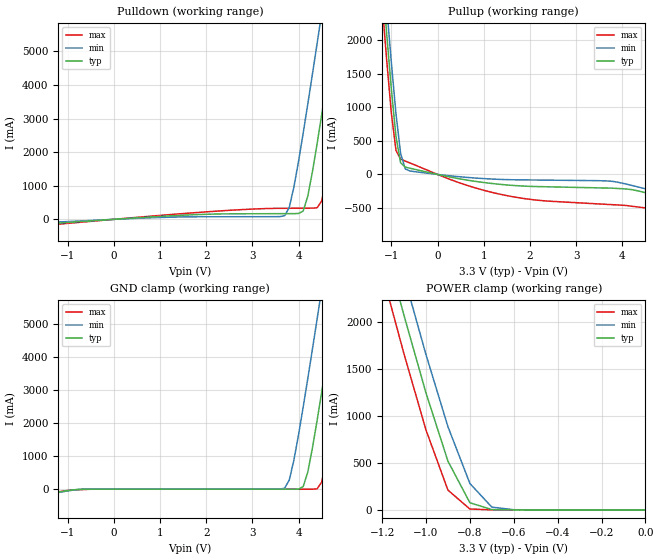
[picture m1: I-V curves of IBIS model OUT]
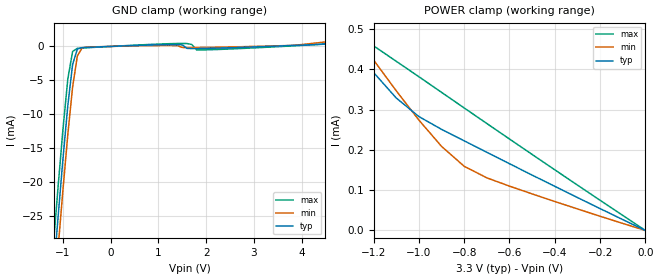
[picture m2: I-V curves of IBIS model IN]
|   TEXAS INSTRUMENTS INCORPORATED
|   Standard Linear and Logic
|   IBIS Model of SN74ALVCH16334
|   16-BIT Universal Bus Driver with 3-state outputs
|   48-pin DGG, DGV, or DL Package
[IBIS Ver]   2.1
[Comment char]  |_char
[File Name]   alvch16334.ibs
[File Rev]   2.0
[Date]   8/1/97
[Source]   File originated at Texas Instruments, Inc.
[Notes]   The following is an IBIS list for the ALVCH16334.
|   - This file may be incomplete or may not be fully compliant
|   with the IBIS specification. It will be replaced with a
|   version that is IBIS Revision 3.2 compliant and is complete
|   and accurate.  Please email all questions and comments to
|   sllibis@ti.com.
|   - All test data contained in this file are derived from
|   hspice(tm) simulations.
|   - File created by Ramzi Ammar, SLL Applications
[Disclaimer]
* Property of Texas Instruments Incorporated.  Unauthorized *
* reproduction and/or distribution is strictly prohibited. *
* This product is protected under copyright law. *
* Created 1997, (C) Copyright 1997, Texas Instruments Inc., *
* All Rights Reserved *
* UNLESS THERE IS A SIGNED, WRITTEN AGREEMENT TO THE *
* CONTRARY, TEXAS INSTRUMENTS ("TI") IS PROVIDING THE IBIS *
* MODELS "AS IS" AND WITHOUT ANY WARRANTY, EXPRESSED OR *
* IMPLIED.  TI assumes no liability for: *
* 1) the accuracy of the IBIS models provided to your *
* company; *
* 2) the proper functioning of these IBIS models in your *
* design or for any resulting applications; or *
* 3) infringement of patents, copyrights or intellectual *
* property rights resulting from your use of these *
* IBIS models. *
* TI provides IBIS Models as a service to our customers. *
* You and your company shall not distribute, sell or give *
* these models to anyone else without prior written *
* permission from TI. *
* TI reserves the right to make changes to our products or *
* to discontinue any semiconductor product or service *
* without notice, and advises our customers to obtain the *
* latest version of relevant information to verify, before *
* placing orders, that the information being relied on is *
* current. *
* Please be aware that your receipt and use of the IBIS *
* information provided shall serve as acceptance of these *
* terms and conditions.  If you do not accept these terms, *
* you should return or destroy the IBIS models and any *
* other accompanying information immediately. *
[Component]   ALVCH16334_DGG
[Manufacturer]  Texas Instruments, Inc.
[Package]
|   typ   min   max
R_pkg   0.056   0.039   0.068
L_pkg   3.39nH   3.078nH   3.995nH
C_pkg   0.52pF   0.414pF   0.668pF
[Pin]   signal_name   model_name   R_pin   L_pin   C_pin
1   OE_BAR   NC   0.039   3.987nH   0.654pF
2   Y1   OUT   0.047   3.725nH   0.659pF
3   Y2   OUT   0.059   3.692nH   0.604pF
4   GND   GND   0.068   3.675nH   0.606pF
5   Y3   OUT   0.055   3.473nH   0.547pF
6   Y4   OUT   0.056   3.402nH   0.497pF
7   VCC   POWER   0.057   3.3nH   0.492pF
8   Y5   OUT   0.056   3.189nH   0.455pF
9   Y6   OUT   0.058   3.154nH   0.449pF
10   GND   GND   0.058   3.094nH   0.436pF
11   Y7   OUT   0.058   3.078nH   0.424pF
12   Y8   OUT   0.06   3.081nH   0.414pF
13   Y9   OUT   0.061   3.097nH   0.416pF
14   Y10   OUT   0.06   3.126nH   0.427pF
15   GND   GND   0.061   3.158nH   0.44pF
16   Y11   OUT   0.058   3.173nH   0.45pF
17   Y12   OUT   0.056   3.189nH   0.455pF
18   VCC   POWER   0.056   3.265nH   0.49pF
19   Y13   OUT   0.054   3.322nH   0.492pF
20   Y14   OUT   0.052   3.388nH   0.544pF
21   GND   GND   0.064   3.591nH   0.605pF
22   Y15   OUT   0.059   3.677nH   0.612pF
23   Y16   OUT   0.046   3.678nH   0.668pF
24   NC   NC   0.041   3.979nH   0.659pF
25   LE_BAR   NC   0.04   3.995nH   0.658pF
26   A16   IN   0.046   3.69nH   0.662pF
27   A15   IN   0.057   3.649nH   0.602pF
28   GND   GND   0.066   3.615nH   0.602pF
29   A14   IN   0.055   3.447nH   0.547pF
30   A13   IN   0.054   3.326nH   0.492pF
31   VCC   POWER   0.055   3.239nH   0.488pF
32   A12   IN   0.056   3.183nH   0.454pF
33   A11   IN   0.057   3.144nH   0.447pF
34   GND   GND   0.058   3.099nH   0.436pF
35   A10   IN   0.059   3.086nH   0.425pF
36   A9   IN   0.06   3.081nH   0.414pF
37   A8   IN   0.061   3.097nH   0.415pF
38   A7   IN   0.06   3.119nH   0.427pF
39   GND   GND   0.06   3.144nH   0.439pF
40   A6   IN   0.056   3.13nH   0.446pF
41   A5   IN   0.057   3.208nH   0.456pF
42   VCC   POWER   0.056   3.247nH   0.487pF
43   A4   IN   0.054   3.328nH   0.491pF
44   A3   IN   0.053   3.413nH   0.546pF
45   GND   GND   0.066   3.609nH   0.606pF
46   A2   IN   0.058   3.689nH   0.607pF
47   A1   IN   0.047   3.727nH   0.662pF
48   CLK   NC   0.04   3.978nH   0.655pF
[Component]   ALVCH16334_DGV
[Manufacturer]  Texas Instruments, Inc.
[Package]
|   typ   min   max
R_pkg   0.063   0.043   0.09
L_pkg   3.077nH   2.377nH   4.305nH
C_pkg   0.387pF   0.281pF   0.565pF
[Pin]   signal_name   model_name   R_pin   L_pin   C_pin
1   OE_BAR   NC   0.082   4.277nH   0.562pF
2   Y1   OUT   0.09   4.02nH   0.554pF
3   Y2   OUT   0.087   3.719nH   0.478pF
4   GND   GND   0.087   3.456nH   0.417pF
5   Y3   OUT   0.076   3.207nH   0.411pF
6   Y4   OUT   0.044   2.929nH   0.39pF
7   VCC   POWER   0.046   2.803nH   0.335pF
8   Y5   OUT   0.047   2.683nH   0.321pF
9   Y6   OUT   0.048   2.579nH   0.311pF
10   GND   GND   0.049   2.505nH   0.302pF
11   Y7   OUT   0.048   2.4nH   0.289pF
12   Y8   OUT   0.051   2.4nH   0.283pF
13   Y9   OUT   0.051   2.4nH   0.283pF
14   Y10   OUT   0.05   2.433nH   0.291pF
15   GND   GND   0.048   2.46nH   0.298pF
16   Y11   OUT   0.048   2.585nH   0.312pF
17   Y12   OUT   0.046   2.652nH   0.319pF
18   VCC   POWER   0.045   2.787nH   0.336pF
19   Y13   OUT   0.046   2.962nH   0.394pF
20   Y14   OUT   0.074   3.208nH   0.409pF
21   GND   GND   0.087   3.488nH   0.417pF
22   Y15   OUT   0.087   3.741nH   0.478pF
23   Y16   OUT   0.089   3.99nH   0.546pF
24   NC   NC   0.084   4.305nH   0.557pF
25   LE_BAR   NC   0.082   4.286nH   0.565pF
26   A16   IN   0.086   3.933nH   0.554pF
27   A15   IN   0.086   3.699nH   0.475pF
28   GND   GND   0.089   3.522nH   0.42pF
29   A14   IN   0.079   3.234nH   0.413pF
30   A13   IN   0.043   2.88nH   0.385pF
31   VCC   POWER   0.045   2.779nH   0.332pF
32   A12   IN   0.045   2.636nH   0.317pF
33   A11   IN   0.047   2.553nH   0.309pF
34   GND   GND   0.048   2.468nH   0.298pF
35   A10   IN   0.05   2.424nH   0.29pF
36   A9   IN   0.05   2.377nH   0.281pF
37   A8   IN   0.05   2.387nH   0.281pF
38   A7   IN   0.05   2.431nH   0.29pF
39   GND   GND   0.048   2.475nH   0.299pF
40   A6   IN   0.048   2.557nH   0.309pF
41   A5   IN   0.047   2.671nH   0.319pF
42   VCC   POWER   0.046   2.804nH   0.334pF
43   A4   IN   0.044   2.935nH   0.39pF
44   A3   IN   0.074   3.203nH   0.412pF
45   GND   GND   0.085   3.444nH   0.416pF
46   A2   IN   0.085   3.723nH   0.477pF
47   A1   IN   0.09   4.012nH   0.547pF
48   CLK   NC   0.083   4.288nH   0.558pF
[Component]   ALVCH16334_DL
[Manufacturer]  Texas Instruments, Inc.
[Package]
|   typ   min   max
R_pkg   0.048   0.038   0.053
L_pkg   6.046nH   5.084nH   7.968nH
C_pkg   0.813pF   0.569pF   1.157pF
[Pin]   signal_name   model_name   R_pin   L_pin   C_pin
1   OE_BAR   NC   0.046   7.968nH   1.017pF
2   Y1   OUT   0.044   7.299nH   1.157pF
3   Y2   OUT   0.043   6.765nH   1.058pF
4   GND   GND   0.041   6.269nH   0.933pF
5   Y3   OUT   0.038   5.856nH   0.829pF
6   Y4   OUT   0.046   5.802nH   0.79pF
7   VCC   POWER   0.05   5.656nH   0.738pF
8   Y5   OUT   0.053   5.5nH   0.643pF
9   Y6   OUT   0.052   5.304nH   0.606pF
10   GND   GND   0.053   5.189nH   0.583pF
11   Y7   OUT   0.051   5.084nH   0.569pF
12   Y8   OUT   0.053   5.862nH   0.833pF
13   Y9   OUT   0.053   5.862nH   0.833pF
14   Y10   OUT   0.051   5.084nH   0.569pF
15   GND   GND   0.053   5.189nH   0.583pF
16   Y11   OUT   0.052   5.304nH   0.606pF
17   Y12   OUT   0.053   5.5nH   0.643pF
18   VCC   POWER   0.05   5.656nH   0.738pF
19   Y13   OUT   0.046   5.802nH   0.79pF
20   Y14   OUT   0.038   5.856nH   0.829pF
21   GND   GND   0.041   6.269nH   0.933pF
22   Y15   OUT   0.043   6.765nH   1.058pF
23   Y16   OUT   0.044   7.299nH   1.157pF
24   NC   NC   0.046   7.968nH   1.017pF
25   LE_BAR   NC   0.046   7.968nH   1.017pF
26   A16   IN   0.044   7.299nH   1.157pF
27   A15   IN   0.043   6.765nH   1.058pF
28   GND   GND   0.041   6.269nH   0.933pF
29   A14   IN   0.038   5.856nH   0.829pF
30   A13   IN   0.046   5.802nH   0.79pF
31   VCC   POWER   0.05   5.656nH   0.738pF
32   A12   IN   0.053   5.5nH   0.643pF
33   A11   IN   0.052   5.304nH   0.606pF
34   GND   GND   0.053   5.189nH   0.583pF
35   A10   IN   0.051   5.084nH   0.569pF
36   A9   IN   0.053   5.862nH   0.833pF
37   A8   IN   0.053   5.862nH   0.833pF
38   A7   IN   0.051   5.084nH   0.569pF
39   GND   GND   0.053   5.189nH   0.583pF
40   A6   IN   0.052   5.304nH   0.606pF
41   A5   IN   0.053   5.5nH   0.643pF
42   VCC   POWER   0.05   5.656nH   0.738pF
43   A4   IN   0.046   5.802nH   0.79pF
44   A3   IN   0.038   5.856nH   0.829pF
45   GND   GND   0.041   6.269nH   0.933pF
46   A2   IN   0.043   6.765nH   1.058pF
47   A1   IN   0.044   7.299nH   1.157pF
48   CLK   NC   0.046   7.967nH   1.017pF
| Models and submodels in the file (2): OUT (3-state), IN (Input)
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|   Model ALVCH16334_OUT
[Model]   OUT
Model_type   3-state
Polarity   Non-Inverting
Enable   Active-High
|Variable   typ   min   max
C_comp   7.0pF   NA   NA
[Voltage range]   3.3   3.0   3.6
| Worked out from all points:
|   slope of the pulldown table from 0 to 0.495 V, typ, clamps not added: 10.9 ohm
|   slope of the pullup table from 0 to 0.495 V, typ, clamps not added: 7.36 ohm
|   GND clamp passes 1 mA (typ) near -0.52 V on its own axis
|   POWER clamp passes 1 mA (typ) near -0.63 V on its own axis
[Pullup]   | Note: Vtable = Vcc - Voutput
|   Voltage   I(typ)   I(min)   I(max)
-3.3V     22.55A     22.92A     22.19A
-1.2V     2.946A     3.36A      2.546A
-1.1V     2.084A     2.494A     1.692A
-1V       1.269A     1.664A     910.2mA
-900mV    565.6mA    903.2mA    357.9mA
-800mV    174.2mA    315.2mA    229.6mA
-700mV    109.9mA    82.5mA     199.4mA
-600mV    92.9mA     51.79mA    171.6mA
1.4V      -150.2mA   -74.75mA   -300.9mA
3.8V      -204.5mA   -103.9mA   -450mA
4.7V      -306mA     -248.4mA   -521.1mA
6.6V      -655.4mA   -587.7mA   -903.7mA
[Pulldown]
|   Voltage   I(typ)   I(min)   I(max)
-3.3V     -415.9mA   -421.8mA   -412.8mA
-1.1V     -104mA     -73.21mA   -132.2mA
3.7V      169.6mA    108.9mA    328.9mA
3.8V      170mA      361.2mA    329.7mA
3.9V      170.6mA    966mA      330.5mA
4.1V      247.2mA    2.567A     332.1mA
4.2V      690.8mA    3.435A     332.9mA
4.4V      2.241A     5.223A     343.5mA
4.5V      3.108A     6.133A     545.3mA
4.8V      5.815A     8.898A     2.861A
5.1V      8.589A     11.69A     5.578A
6.6V      22.73A     25.85A     19.7A
[POWER_Clamp]   | Note: Vtable = Vcc - Voutput
|   Voltage   I(typ)   I(min)   I(max)
-3.3V     22.55A     22.92A     22.19A
-1.2V     2.935A     3.354A     2.523A
-1.1V     2.069A     2.487A     1.659A
-1V       1.245A     1.653A     850.2mA
-900mV    518.9mA    885.7mA    209.9mA
-800mV    75.78mA    281.1mA    8.953mA
-700mV    2.801mA    29.05mA    160uA
-600mV    75.4uA     1.568mA    1.514uA
0V        990pA      903.2pA    1.08nA
[GND_Clamp]
|   Voltage   I(typ)   I(min)   I(max)
-3.3V     -640.3mA   -651.6mA   -629.4mA
-800mV    -11.24mA   -14.93mA   -17.28mA
3.7V      58.53nA    29.05mA    1.13nA
3.9V      75.43uA    885.7mA    1.234nA
4.1V      75.77mA    2.487A     22.94nA
4.2V      518.9mA    3.354A     1.514uA
4.4V      2.069A     5.142A     8.953mA
4.5V      2.935A     6.052A     209.9mA
4.8V      5.64A      8.816A     2.523A
5.1V      8.413A     11.61A     5.238A
5.2V      9.345A     12.55A     6.161A
6.6V      22.55A     25.76A     19.34A
[Ramp]
| variable   typ   min   max
dV/dt_r   1.7364E+00/1.9231E-10  1.3957E+00/2.9903E-10  2.0142E+00/1.7016E-10
dV/dt_f   1.6302E+00/2.0099E-10  1.3593E+00/4.4330E-10  1.8600E+00/1.6534E-10
|   Model ALVCH16334_IN
[Model]   IN
Model_type   Input
Polarity   Non-Inverting
Vinl = 0.8V
Vinh = 2.0V
|Variable   typ   min   max
C_comp   6pF   NA   NA
[Voltage Range]   3.3   3.0   3.6
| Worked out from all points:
|   GND clamp passes 1 mA (typ) near -0.73 V on its own axis
|   POWER clamp passes 1 mA (typ) near -1.97 V on its own axis
[POWER_Clamp]   | Note: Vtable = Vcc - Voutput
|   Voltage   I(typ)   I(min)   I(max)
-3.3V     2.121mA    2.168mA    2.076mA
-1.4V     540.7uA    581.6uA    541.7uA
-1.3V     464.2uA    501.6uA    497.2uA
-1.2V     392uA      423uA      458.1uA
-1.1V     328.8uA    346.6uA    419.8uA
-1V       282.6uA    273.9uA    381.5uA
-900mV    250.9uA    208.7uA    342.7uA
-800mV    222.4uA    159.2uA    304uA
-700mV    193.9uA    130.6uA    265.4uA
-600mV    165.6uA    110uA      226.9uA
-300mV    81.7uA     53.43uA    112.6uA
0V        1.064nA    1.048nA    1.063nA
[GND_Clamp]
|   Voltage   I(typ)   I(min)   I(max)
-3.3V     -228.9mA   -233.1mA   -224.8mA
-1.2V     -33.4mA    -38.07mA   -28.95mA
-1.1V     -24.73mA   -29.35mA   -20.28mA
-1V       -16.38mA   -20.91mA   -12.02mA
-900mV    -8.673mA   -12.94mA   -4.776mA
-800mV    -2.646mA   -5.969mA   -744.8uA
-700mV    -380.8uA   -1.394mA   -282.9uA
-600mV    -177.8uA   -207.9uA   -234.2uA
-500mV    -142.4uA   -98.01uA   -194.6uA
1.4V      255.6uA    108.4uA    429uA
3.8V      137.4uA    159.2uA    74.84uA
6.6V      2.121mA    2.422mA    1.823mA
